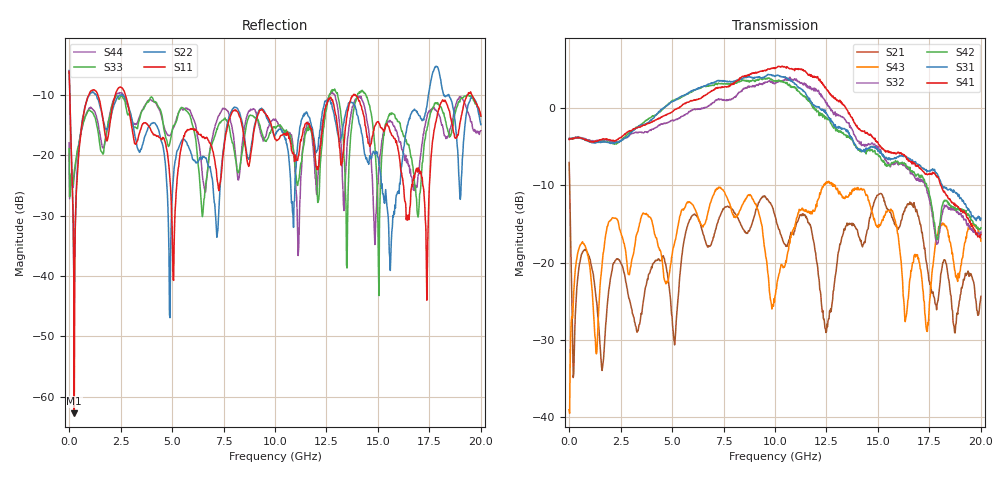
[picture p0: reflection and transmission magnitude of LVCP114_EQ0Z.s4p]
!Agilent Technologies,N5230A,MY46400459,A.07.50.48
!Agilent N5230A: A.07.50.48
!Date: Monday, January 09, 2012 14:00:16
!Correction: S11(Full 4 Port(1,2,3,4))
!S12(Full 4 Port(1,2,3,4))
!S13(Full 4 Port(1,2,3,4))
!S14(Full 4 Port(1,2,3,4))
!S21(Full 4 Port(1,2,3,4))
!S22(Full 4 Port(1,2,3,4))
!S23(Full 4 Port(1,2,3,4))
!S24(Full 4 Port(1,2,3,4))
!S31(Full 4 Port(1,2,3,4))
!S32(Full 4 Port(1,2,3,4))
!S33(Full 4 Port(1,2,3,4))
!S34(Full 4 Port(1,2,3,4))
!S41(Full 4 Port(1,2,3,4))
!S42(Full 4 Port(1,2,3,4))
!S43(Full 4 Port(1,2,3,4))
!S44(Full 4 Port(1,2,3,4))
!S4P File: Measurements: <S11,S12,S13,S14>,
!<S21,S22,S23,S24>,
!<S31,S32,S33,S34>,
!<S41,S42,S43,S44>:
# Hz S  dB  R 50
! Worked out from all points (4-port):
!   801 points, 300 kHz to 20 GHz, reference 50 ohm
!   strongest paths, dB at 300 kHz, 5 GHz, 10 GHz, 15 GHz, 20 GHz:
!     S41: -4.1, -0.5, 5.1, -4.5, -16.4
!     S31: -4.0, 0.8, 4.1, -5.6, -14.3
!     S42: -4.0, 0.9, 3.5, -6.0, -15.5
!     S32: -3.9, -1.6, 3.2, -5.2, -16.1
!     S43: -39.1, -19.0, -24.3, -15.2, -17.2
!     S21: -7.1, -27.0, -14.0, -11.3, -24.4
!   lowest |S11| = -62.7 dB at 250.3 MHz (marker M1), VSWR 1.00, Z = 50.1 - j0.0514 ohm
!   |S11| at or under -10 dB: 34.39 MHz to 952.8 MHz (918.4 MHz wide, 186 % of centre); 2.735 GHz to 13.8 GHz (11.07 GHz wide, 134 % of centre); 13.91 GHz to 19.35 GHz (5.438 GHz wide, 32.7 % of centre)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
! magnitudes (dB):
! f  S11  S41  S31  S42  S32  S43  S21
! 300 kHz  -6.1  -4.1  -4.0  -4.0  -3.9  -39.1  -7.1
! 250.3 MHz  -62.7  -3.9  -3.9  -3.9  -3.9  -22.7  -31.5
! 1.125 GHz  -9.2  -4.4  -4.5  -4.4  -4.3  -23.8  -21.0
! 4.9 GHz  -23.9  -0.7  0.7  0.7  -1.7  -20.8  -24.2
! 8.025 GHz  -12.5  3.3  3.5  3.3  1.4  -14.0  -13.6
! 15.6 GHz  -16.2  -5.8  -6.7  -7.4  -7.6  -13.3  -13.5
! 20 GHz  -13.5  -16.4  -14.3  -15.5  -16.1  -17.2  -24.4
